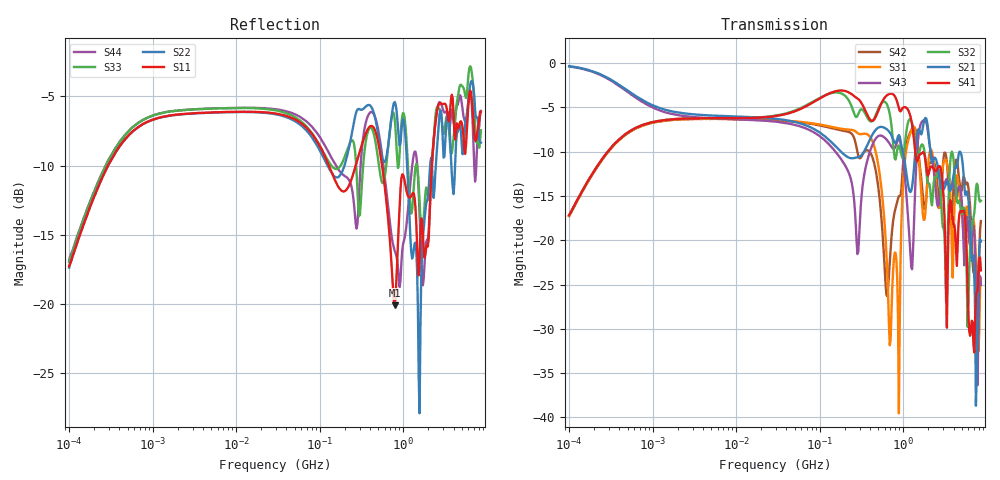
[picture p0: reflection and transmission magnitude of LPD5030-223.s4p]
# MHz S MA R 50
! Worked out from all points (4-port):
!   498 points, 100 kHz to 8.5 GHz, reference 50 ohm
!   strongest paths, dB at 100 kHz, 1.698 MHz, 29.49 MHz, 500.7 MHz, 8.5 GHz:
!     S41: -17.2, -6.4, -6.0, -5.4, -23.4
!     S21: -0.3, -5.4, -6.3, -7.3, -20.2
!     S32: -17.2, -6.3, -5.9, -5.2, -15.5
!     S43: -0.4, -5.7, -6.6, -8.3, -25.0
!     S31: -17.3, -6.4, -6.4, -11.4, -24.3
!     S42: -17.3, -6.4, -6.5, -13.9, -17.8
!   lowest |S11| = -20.1 dB at 790.5 MHz (marker M1), VSWR 1.22, Z = 45.6 - j8.41 ohm
!   |S11| at or under -10 dB: start of sweep to 291.7 kHz; 128.8 MHz to 269.5 MHz (140.7 MHz wide, 70.6 % of centre); 557.9 MHz to 2.198 GHz (1.64 GHz wide, 119 % of centre)
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0.1  0.1369 71.7  0.9611 -7.9  0.1371 -106.8  0.1385 73.3
     0.9611 -7.9  0.1355 71.9  0.1381 73.3  0.1372 -106.8
     0.1371 -106.8  0.1381 73.3  0.1418 70.9  0.9581 -8.2
     0.1385 73.3  0.1372 -106.8  0.9581 -8.2  0.1439 71.7
142.5721  0.2937 -39.3  0.353 -103.5  0.4354 71.0  0.6862 -17.6
          0.353 -103.5  0.2945 -25.1  0.6801 -22.7  0.4277 72.9
          0.4354 71.0  0.6801 -22.7  0.3124 -29.3  0.3307 -107.5
          0.6862 -17.6  0.4277 72.9  0.3307 -107.5  0.3319 -38.9
790.5161  0.09911 -112.8  0.3556 -62.8  0.08519 -49.0  0.652 -135.0
          0.3556 -62.8  0.5358 -126.0  0.2897 -144.5  0.1454 -12.2
          0.08519 -49.0  0.2897 -144.5  0.4653 -117.8  0.3311 -63.1
          0.652 -135.0  0.1454 -12.2  0.3311 -63.1  0.1558 -127.5
1568.416  0.1468 164.6  0.4178 -177.4  0.2544 135.0  0.3043 108.8
          0.4178 -177.4  0.0404 165.8  0.321 122.1  0.2701 140.5
          0.2544 135.0  0.321 122.1  0.2337 127.7  0.4271 -152.5
          0.3043 108.8  0.2701 140.5  0.4271 -152.5  0.2131 122.9
5634.932  0.3735 5.9  0.1811 -43.4  0.1433 -24.2  0.1116 -80.6
          0.1811 -43.4  0.4653 4.3  0.1054 -93.4  0.2067 -48.2
          0.1433 -24.2  0.1054 -93.4  0.5542 -6.8  0.1167 -4.4
          0.1116 -80.6  0.2067 -48.2  0.1167 -4.4  0.4485 -5.7
6764.496  0.5005 -158.6  0.07719 162.3  0.1297 174.8  0.03454 151.8
          0.07719 162.3  0.6327 -170.2  0.1257 -100.9  0.07413 137.6
          0.1297 174.8  0.1257 -100.9  0.6478 -177.4  0.1159 -163.2
          0.03454 151.8  0.07413 137.6  0.1159 -163.2  0.4596 -177.3
8500  0.4942 -39.3  0.09819 19.8  0.06069 1.8  0.06764 38.8
      0.09819 19.8  0.3822 -58.8  0.1671 0.4  0.1284 -4.4
      0.06069 1.8  0.1671 0.4  0.4237 -40.9  0.05592 22.0
      0.06764 38.8  0.1284 -4.4  0.05592 22.0  0.498 -41.8
